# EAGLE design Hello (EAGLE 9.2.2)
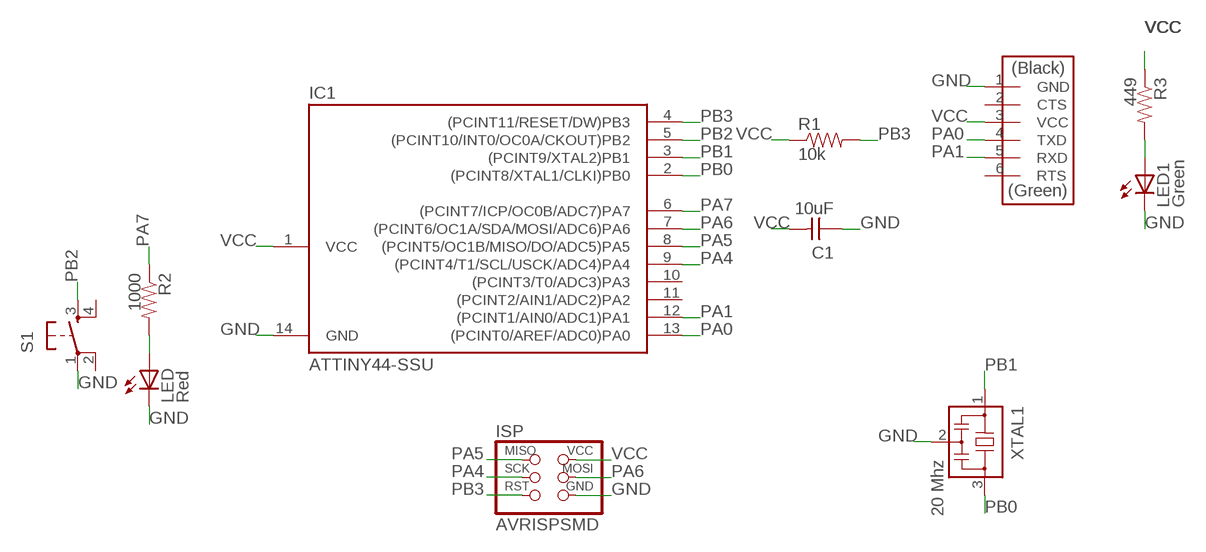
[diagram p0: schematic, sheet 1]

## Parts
C1  10uF  CAP-UNPOLARIZEDFAB  [C1206FAB]
FTDI  FTDI-SMD-HEADER  [1X06SMD]
IC1  ATTINY44-SSU  [SOIC14]
ISP  AVRISPSMD  [2X03SMD]
LED  Red  LEDFAB1206  [LED1206FAB]
LED1  Green  LEDFAB1206  [LED1206FAB]
R1  10k  RESISTOR1206  [1206]
R2  1000  RESISTOR1206  [1206]
R3  449  RESISTOR1206  [1206]
S1  6MM_SWITCH6MM_SWITCH  [6MM_SWITCH]
XTAL1  20 Mhz  RESONATOR  [EFOBM]

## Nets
GND: C1.1 FTDI.1(GND) IC1.14(GND) ISP.6(GND) LED1.2(C) LED.2(C) S1.1(P) XTAL1.2
N$1: LED.1(A) R2.2
N$2: LED1.1(A) R3.2
PA0: FTDI.4(TXD) IC1.13((PCINT0/AREF/ADC0)PA0)
PA1: FTDI.5(RXD) IC1.12((PCINT1/AIN0/ADC1)PA1)
PA4: IC1.9((PCINT4/T1/SCL/USCK/ADC4)PA4) ISP.3(SCK)
PA5: IC1.8((PCINT5/OC1B/MISO/DO/ADC5)PA5) ISP.1(MISO)
PA6: IC1.7((PCINT6/OC1A/SDA/MOSI/ADC6)PA6) ISP.4(MOSI)
PA7: IC1.6((PCINT7/ICP/OC0B/ADC7)PA7) R2.1
PB0: IC1.2((PCINT8/XTAL1/CLKI)PB0) XTAL1.3
PB1: IC1.3((PCINT9/XTAL2)PB1) XTAL1.1
PB2: IC1.5((PCINT10/INT0/OC0A/CKOUT)PB2) S1.3(S)
PB3: IC1.4((PCINT11/RESET/DW)PB3) ISP.5(RST) R1.2
VCC: C1.2 FTDI.3(VCC) IC1.1(VCC) ISP.2(VCC) R1.1 R3.1
Unconnected: FTDI.2(CTS) FTDI.6(RTS) IC1.10((PCINT3/T0/ADC3)PA3) IC1.11((PCINT2/AIN1/ADC2)PA2) S1.2(P1) S1.4(S1)

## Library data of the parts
C1 = fab:CAP-UNPOLARIZED
FTDI = fab:FTDI-SMD-HEADER
IC1 = fab:ATTINY44
ISP = fab:AVRISP
LED LED1 = fab:LED: LED
R1-R3 = SparkFun-Resistors:RESISTOR: Generic Resistor Package
S1 = fab:6MM_SWITCH: OMRON SWITCH
XTAL1 = fab:RESONATOR

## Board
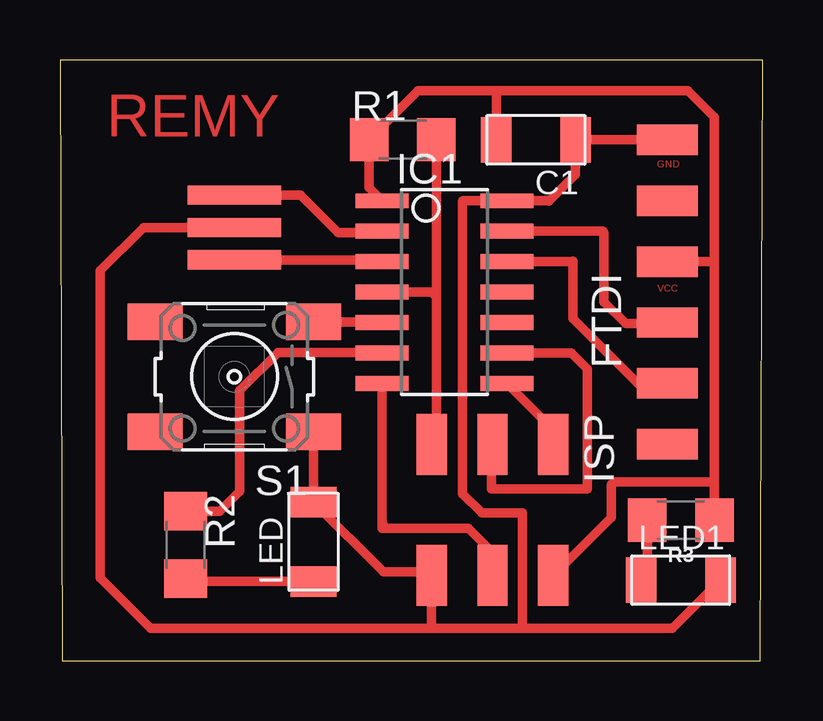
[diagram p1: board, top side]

Size 29.3 x 25.06 mm. Coordinates in mm from the lower left corner, seen from the top.
Outline: 0.1,0 29.2,0 29.3,25.06 0,25.06 0.1,0
Copper layers (1*16): Top 0.035mm / dielectric 1.5mm / Bottom 0.035mm
Design rules "default *": minimum track width 0.4mm, minimum drill 0.4mm, track to track 0.3mm, track to pad 0.3mm, pad to pad 0.3mm, via to via 6mil, smd to smd 0.3mm, copper to edge 40mil, drill to drill 6mil, minimum pad ring 10mil, minimum via ring 8mil, stop-mask expansion 4mil, vias tented up to drill 0mil, thermal gap 10mil

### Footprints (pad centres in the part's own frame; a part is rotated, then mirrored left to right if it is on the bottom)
C1206FAB = smd 1.27 x 1.905: 1 -1.651,0; 2 1.651,0
1X06SMD = smd 2.54 x 1.27: 1 0,6.35; 2 0,3.81; 3 0,1.27; 4 0,-1.27; 5 0,-3.81; 6 0,-6.35
SOIC14 = smd 0.61 x 2.21: 1 -3.81,-2.603; 2 -2.54,-2.603; 3 -1.27,-2.603; 4 0,-2.603; 5 1.27,-2.603; 6 2.54,-2.603; 7 3.81,-2.603; 8 3.81,2.603; 9 2.54,2.603; 10 1.27,2.603; 11 0,2.603; 12 -1.27,2.603; 13 -2.54,2.603; 14 -3.81,2.603
2X03SMD = smd 2.54 x 1.27: 1 -2.54,2.54; 2 2.92,2.54; 3 -2.54,0; 4 2.92,0; 5 -2.54,-2.54; 6 2.92,-2.54
LED1206FAB = smd 1.27 x 1.905: 1 -1.651,0; 2 1.651,0
1206 = smd 1.6 x 1.8: 1 -1.4,0; 2 1.4,0
6MM_SWITCH = smd 2.286 x 1.524: 1 -3.302,2.286; 2 3.302,2.286; 3 -3.302,-2.286; 4 3.302,-2.286
EFOBM = smd 0.8 x 3.9: 1 -1.35,0; 2 0,0; 3 1.35,0

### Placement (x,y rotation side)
C1  19.84,21.73 180 top
FTDI  25.32,15.38 0 top
IC1  16.03,15.38 270 top
ISP  18.03,6.49 270 top
LED  10.57,4.97 90 top
LED1  25.88,3.37 0 top
R1  14.29,21.73 0 top
R2  5.24,4.84 270 top
R3  25.88,5.87 180 top
S1  7.27,11.85 180 top
XTAL1  7.27,18.08 90 top

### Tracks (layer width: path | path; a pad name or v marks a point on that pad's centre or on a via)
GND
  Top 0.4: XTAL1.2 3.49,18.08 1.68,16.27 1.68,3.47 3.78,1.37 15.48,1.37 | S1.1 LED.2 13.48,3.71 15.36,3.71 ISP.6 | 15.49,2.68 15.49,3.27 | 15.49,3.27 ISP.6 | IC1.14 20.36,19.19 20.38,19.17 21.49,20.28 C1.1 FTDI.1 | 18.52,19.07 IC1.14 | 15.48,3.27 15.49,3.27 | 15.48,1.37 19.28,1.37 | 19.28,1.37 25.53,1.37 LED1.2 | ISP.6 15.49,1.38 15.48,1.37 | IC1.14 16.8,19.19 16.78,19.17 16.78,6.97 17.58,6.17 19.28,6.17 19.28,1.37
N$1
  Top 0.4: R2.2 5.36,3.32 LED.1
N$2
  Top 0.4: R3.2 24.48,3.62 LED1.1
PA0
  Top 0.4: IC1.13 22.63,17.92 22.68,17.87 22.68,14.97 23.58,14.07 25.28,14.07 FTDI.4
PA1
  Top 0.4: IC1.12 21.36,16.65 21.38,16.67 21.38,14.27 24.08,11.57 FTDI.5
PA4
  Top 0.152: ISP.3
  Top 0.4: ISP.3 17.98,8.99 17.98,7.17 21.98,7.17 21.98,12.17 21.31,12.84 IC1.9
PA5
  Top 0.4: ISP.1 20.57,9.64 IC1.8
PA6
  Top 0.4: IC1.7 13.43,5.73 | 13.43,5.73 13.43,5.53 17.03,5.53 18.03,4.52 ISP.4 | 13.43,5.73 13.48,5.67
PA7
  Top 0.4: R2.1 6.65,6.24 7.48,7.07 7.48,11.27 9.08,12.87 13.4,12.87 IC1.6
PB0
  Top 0.4: XTAL1.3 10.03,19.43 11.58,17.87 13.38,17.87 IC1.2
PB1
  Top 0.4: XTAL1.1 13.36,16.73 IC1.3
PB2
  Top 0.4: S1.3 13.4,14.14 IC1.5
PB3
  Top 0.4: ISP.5 15.69,9.24 15.69,15.17 | 13.54,15.27 IC1.4 15.48,15.38 15.69,15.17 | R1.2 15.69,15.17
VCC
  Top 0.4: IC1.1 12.89,19.73 R1.1 14.93,23.77 18.28,23.77 | 27.28,16.67 27.28,22.67 26.18,23.77 18.28,23.77 | 27.28,16.67 27.26,16.65 FTDI.3 | C1.2 18.19,23.68 18.28,23.77 | 27.28,16.67 27.28,7.47 | 27.28,7.47 R3.1 | ISP.2 22.98,5.99 22.98,7.37 23.08,7.47 27.28,7.47

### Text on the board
Top: REMY | GND | VCC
